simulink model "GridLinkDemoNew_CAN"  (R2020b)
settings: Solver=FixedStepDiscrete  StartTime=0.0  StopTime=inf  RelTol=1e-3  EnableMultiTasking=on
InitFcn:
  | INNER_PWM=1000
  | OUTER_PWM=50000
undefined symbols (not defined in the file): A, ADCIN0, ADCIN1, ADCINA0, ADCINB0, bit, Compare, conversion, CounterCut_Outer, DCAEVT1, DCAEVT1FILT, Digital, Down, ended, Event, Filtered, GPTRIP1SEL, GPTRIP2SEL, hex2dec, identifier, input, Module, Newinv, of, Single, SPS_EMT_TAPAS_2018b, Standard, start, Tmod1, Trip, TZ1, TZ2, U_dc, Up, version, Zone
libraries: tiiqmathlib x63, c2802xlib x31, c2837xDlib x5, c280xlib x5, c28xdmclib x2, simulink x2, svdutilitieslib x1, c2000lib x1, canmsglib x1
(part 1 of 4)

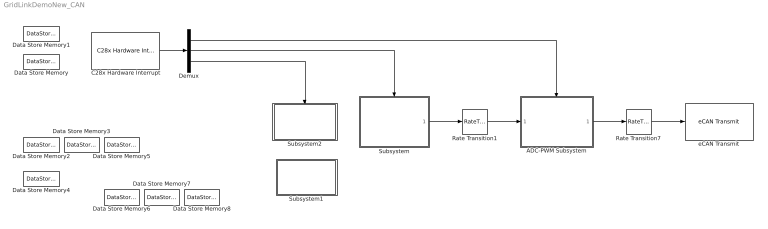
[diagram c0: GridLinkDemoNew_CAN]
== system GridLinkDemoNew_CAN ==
  ADC-PWM Subsystem : Subsystem  TreatAsAtomicUnit=on
  C28x Hardware Interrupt : c2000lib/Scheduling/C28x Hardware Interrupt  irqnumbers=[1 9 3]  pienumbers=[1 7 8]  irqpriorities=[30 10 20]  irqpreempts=[1 1 0]  showinput=off  dspchiptype=C280X
  Data Store Memory : DataStoreMemory  DataStoreName=Counter  ReadBeforeWriteMsg=warning  WriteAfterWriteMsg=warning  WriteAfterReadMsg=warning  ShowAdditionalParam=off
  Data Store Memory1 : DataStoreMemory  DataStoreName=CounterCut  ReadBeforeWriteMsg=warning  WriteAfterWriteMsg=warning  WriteAfterReadMsg=warning  InitialValue=2222  ShowAdditionalParam=off
  Data Store Memory2 : DataStoreMemory  DataStoreName=I_o_A  ReadBeforeWriteMsg=warning  WriteAfterWriteMsg=warning  WriteAfterReadMsg=warning  ShowAdditionalParam=off
  Data Store Memory3 : DataStoreMemory  DataStoreName=I_o_B  ReadBeforeWriteMsg=warning  WriteAfterWriteMsg=warning  WriteAfterReadMsg=warning  ShowAdditionalParam=off
  Data Store Memory4 : DataStoreMemory  DataStoreName=Temp_P1  ReadBeforeWriteMsg=warning  WriteAfterWriteMsg=warning  WriteAfterReadMsg=warning  ShowAdditionalParam=off
  Data Store Memory5 : DataStoreMemory  DataStoreName=I_o_C  ReadBeforeWriteMsg=warning  WriteAfterWriteMsg=warning  WriteAfterReadMsg=warning  ShowAdditionalParam=off
  Data Store Memory6 : DataStoreMemory  DataStoreName=I_s_A  ReadBeforeWriteMsg=warning  WriteAfterWriteMsg=warning  WriteAfterReadMsg=warning  ShowAdditionalParam=off
  Data Store Memory7 : DataStoreMemory  DataStoreName=I_s_B  ReadBeforeWriteMsg=warning  WriteAfterWriteMsg=warning  WriteAfterReadMsg=warning  ShowAdditionalParam=off
  Data Store Memory8 : DataStoreMemory  DataStoreName=I_s_C  ReadBeforeWriteMsg=warning  WriteAfterWriteMsg=warning  WriteAfterReadMsg=warning  ShowAdditionalParam=off
  Demux : Demux  Outputs=3
  Rate Transition1 : RateTransition  Deterministic=off
  Rate Transition7 : RateTransition  Deterministic=off  OutPortSampleTime=0.01
  Subsystem : Subsystem
  Subsystem1 : Subsystem
  Subsystem2 : Subsystem
  eCAN Transmit : c280xlib/eCAN Transmit  chipFamily=C280x  useModule=eCAN_B  mailboxNo=1  messageID=hex2dec('0x01B')  messageType=Standard (11-bit identifier)  enableBlockingMode=on  postInterrupt=off  interruptLine=0
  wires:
  Rate Transition1/1 -> ADC-PWM Subsystem/1(In1)
  ADC-PWM Subsystem/1(Out1) -> Rate Transition7/1
  Subsystem/1(Out3) -> Rate Transition1/1
  C28x Hardware Interrupt/1 -> Demux/1
  Rate Transition7/1 -> eCAN Transmit/1
  Demux/3 -> Subsystem2/Trigger
  Demux/2 -> Subsystem/Trigger
  Demux/1 -> ADC-PWM Subsystem/Trigger
